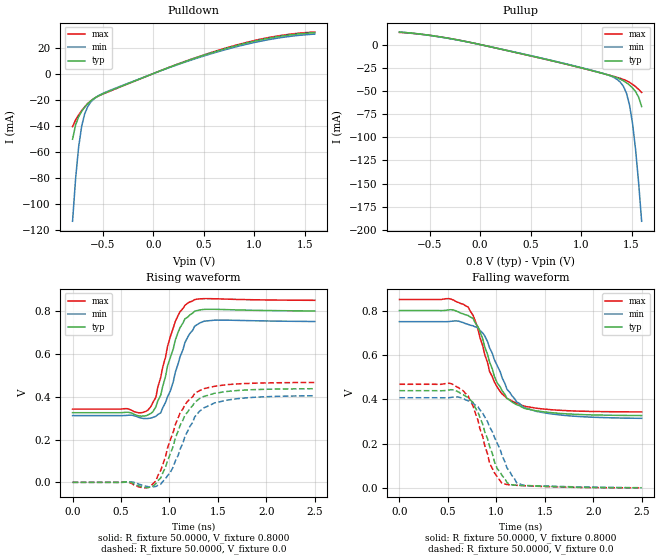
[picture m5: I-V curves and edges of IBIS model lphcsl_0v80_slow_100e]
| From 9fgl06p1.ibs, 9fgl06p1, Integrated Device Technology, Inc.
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[Model]   lphcsl_0v80_slow_100e
Model_type Output
Polarity   Non-Inverting
Enable   Active-High
Vmeas =  0.4000V
Cref =   2.0000pF
Rref =   0.0
Vref =   0.4000V
C_comp   1.1000pF   1.0000pF   1.2000pF
[Temperature Range]   25.0000   85.0000   -40.0
[Voltage Range]   0.8000V   0.7500V   0.8500V
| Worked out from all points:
|   slope of the pulldown table from 0 to 0.12 V, typ, clamps not added: 33 ohm
|   slope of the pullup table from 0 to 0.12 V, typ, clamps not added: 41.5 ohm
|   rising waveform, R_fixture 50.0000, V_fixture 0.8000: 20-80 % time 177ps typ, 191ps min, 178ps max; typ from 0.325 V to 0.801 V
|   rising waveform, R_fixture 50.0000, V_fixture 0.0: 20-80 % time 251ps typ, 249ps min, 239ps max; typ from 0 V to 0.438 V
|   falling waveform, R_fixture 50.0000, V_fixture 0.8000: 20-80 % time 258ps typ, 285ps min, 240ps max; typ from 0.8 V to 0.326 V
|   falling waveform, R_fixture 50.0000, V_fixture 0.0: 20-80 % time 211ps typ, 250ps min, 198ps max; typ from 0.438 V to 0 V
[Pulldown]
|Voltage   I(typ)   I(min)   I(max)
-800mV    -50.49mA   -113.6mA   -40.8mA
-770mV    -39.55mA   -80.95mA   -35.68mA
-740mV    -33.26mA   -56.57mA   -31.82mA
-710mV    -29.08mA   -40.53mA   -28.49mA
-680mV    -25.88mA   -31mA      -25.57mA
-650mV    -23.24mA   -25.46mA   -23.06mA
-590mV    -19.29mA   -19.6mA    -19.31mA
-470mV    -14.59mA   -14.21mA   -14.8mA
40mV      1.232mA    1.183mA    1.259mA
670mV     18.16mA    17.43mA    18.53mA
1.15V     27.29mA    26.19mA    27.81mA
1.6V      31.44mA    30.38mA    31.95mA
[Pullup]
|Voltage   I(typ)   I(min)   I(max)
-800mV    13.44mA    13.49mA    13.08mA
-350mV    7.452mA    7.282mA    7.462mA
220mV     -5.319mA   -5.18mA    -5.366mA
1.12V     -28.48mA   -28.19mA   -28.45mA
1.36V     -36.01mA   -37.85mA   -35.5mA
1.42V     -39.11mA   -45.18mA   -37.65mA
1.45V     -41.2mA    -52.6mA    -39.04mA
1.48V     -43.73mA   -65.24mA   -40.76mA
1.51V     -46.79mA   -85.21mA   -42.88mA
1.54V     -50.76mA   -113.3mA   -45.41mA
1.57V     -56.68mA   -148.9mA   -48.33mA
1.6V      -66.84mA   -190.6mA   -51.65mA
[Ramp]
| variable   typ   min   max
dV/dt_r  0.2626/0.2459n   0.2429/0.2731n   0.2800/0.2326n
dV/dt_f  0.2842/0.2486n   0.2617/0.2798n   0.3044/0.2331n
R_load = 50.0000
[Rising Waveform]
R_fixture= 50.0000
V_fixture= 0.8000
V_fixture_min= 0.7500
V_fixture_max= 0.8500
|time   V(typ)   V(min)   V(max)
0s        325.4mV    311.9mV    342.2mV
780ps     315.3mV    298.6mV    338.8mV
860ps     353.2mV    308.6mV    397.6mV
910ps     407.7mV    324.8mV    490.8mV
1.01ns    584.5mV    428.1mV    682.3mV
1.06ns    664.3mV    513.1mV    751.5mV
1.16ns    763.9mV    653.3mV    827.1mV
1.26ns    800mV      729.4mV    854.1mV
1.46ns    808.5mV    757.8mV    857.9mV
2.5ns     801mV      751.7mV    850.7mV
[Rising Waveform]
R_fixture= 50.0000
V_fixture= 0.0
V_fixture_min= 0.0
V_fixture_max= 0.0
|time   V(typ)   V(min)   V(max)
0s        0V         0V         0V
610ps     -1.204mV   2.029mV    -5.1mV
810ps     -21.38mV   -21.78mV   -15.76mV
910ps     20.81mV    -9.258mV   55.61mV
1.01ns    134.5mV    47.04mV    199.5mV
1.11ns    265.9mV    155.3mV    324.4mV
1.26ns    373mV      305.2mV    414.4mV
1.36ns    402.3mV    349.3mV    438.2mV
1.74ns    430.3mV    392.9mV    461mV
2.5ns     437.6mV    404.8mV    466.7mV
[Falling Waveform]
R_fixture= 50.0000
V_fixture= 0.8000
V_fixture_min= 0.7500
V_fixture_max= 0.8500
|time   V(typ)   V(min)   V(max)
0s        800mV      750mV      850mV
510ps     802.9mV    750.2mV    853.9mV
710ps     777.5mV    737.5mV    815.4mV
810ps     727.6mV    721.9mV    717.6mV
880ps     636.8mV    686mV      602.4mV
980ps     502.6mV    578.1mV    477.4mV
1.11ns    403.5mV    444.7mV    403.3mV
1.21ns    375mV      387.7mV    380.8mV
1.54ns    340.4mV    335.3mV    353.5mV
2.5ns     326.3mV    313.8mV    342.7mV
[Falling Waveform]
R_fixture= 50.0000
V_fixture= 0.0
V_fixture_min= 0.0
V_fixture_max= 0.0
|time   V(typ)   V(min)   V(max)
0s        438.5mV    406.7mV    467.4mV
510ps     441.6mV    406.8mV    472.1mV
660ps     420.6mV    402.8mV    437.5mV
760ps     385.7mV    381.8mV    368.8mV
860ps     286.4mV    336.7mV    230.9mV
930ps     188.1mV    275.3mV    112.9mV
1.06ns    55.51mV    144.6mV    19.62mV
1.21ns    11.74mV    22.79mV    11.66mV
1.29ns    10.33mV    11.05mV    9.949mV
2.5ns     465.9uV    921.7uV    276.7uV
